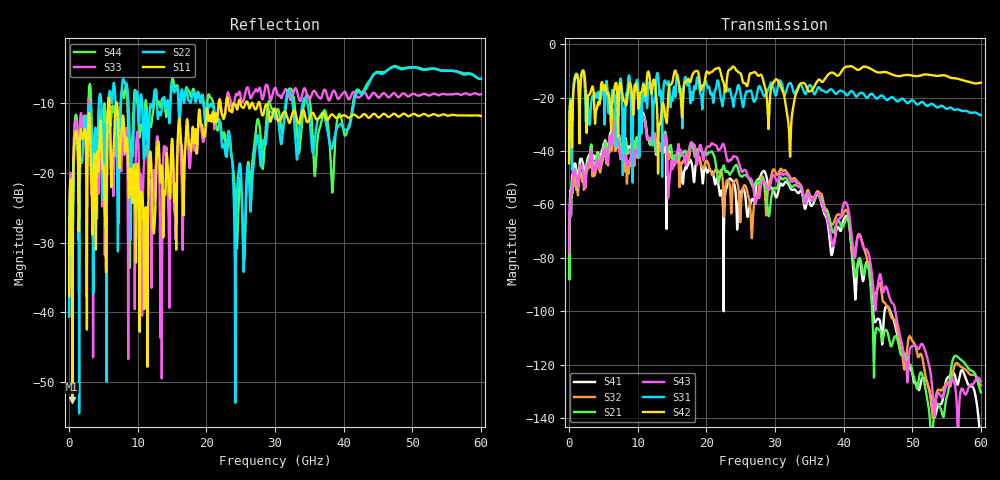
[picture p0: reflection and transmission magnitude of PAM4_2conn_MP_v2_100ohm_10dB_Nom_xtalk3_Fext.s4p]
! Info: Touchstone file created by Circ.  Input file=FAB50GbE_2conn_Midplane_Examax_Topo2_v2_100ohm_10dB_Nom.circ
# Hz S RI R 50
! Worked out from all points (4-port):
!   6000 points, 10 MHz to 60 GHz, reference 50 ohm
!   strongest paths, dB at 10 MHz, 15.01 GHz, 30.01 GHz, 45.01 GHz, 60 GHz:
!     S42: -44.6, -14.5, -13.5, -10.6, -14.4
!     S31: -43.6, -20.6, -18.7, -20.2, -26.5
!     S43: -78.4, -44.2, -49.8, -89.4, -126.3
!     S21: -64.7, -41.7, -54.0, -106.8, -130.4
!     S32: -69.2, -41.7, -47.6, -90.9, -127.8
!     S41: -68.5, -42.8, -56.5, -102.8, -150.1
!   lowest |S11| = -52.6 dB at 480 MHz (marker M1), VSWR 1.00, Z = 50.2 - j0.111 ohm
!   |S11| at or under -10 dB: start of sweep to 5.692 GHz; 6.989 GHz to 21.8 GHz (14.81 GHz wide, 103 % of centre); 27.78 GHz to end of sweep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
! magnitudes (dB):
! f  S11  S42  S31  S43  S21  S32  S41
! 10 MHz  -37.7  -44.6  -43.6  -78.4  -64.7  -69.2  -68.5
! 480 MHz  -52.6  -30.0  -27.2  -52.6  -51.4  -55.2  -49.4
! 10.82 GHz  -26.1  -15.4  -14.6  -27.2  -26.7  -28.3  -25.9
! 14.61 GHz  -22.6  -15.4  -15.5  -52.0  -38.6  -42.3  -39.9
! 22.45 GHz  -12.2  -13.9  -21.9  -37.3  -45.8  -54.3  -62.7
! 32.15 GHz  -12.8  -39.0  -14.6  -50.3  -52.4  -49.5  -53.4
! 60 GHz  -11.8  -14.4  -26.5  -126.3  -130.4  -127.8  -150.1
